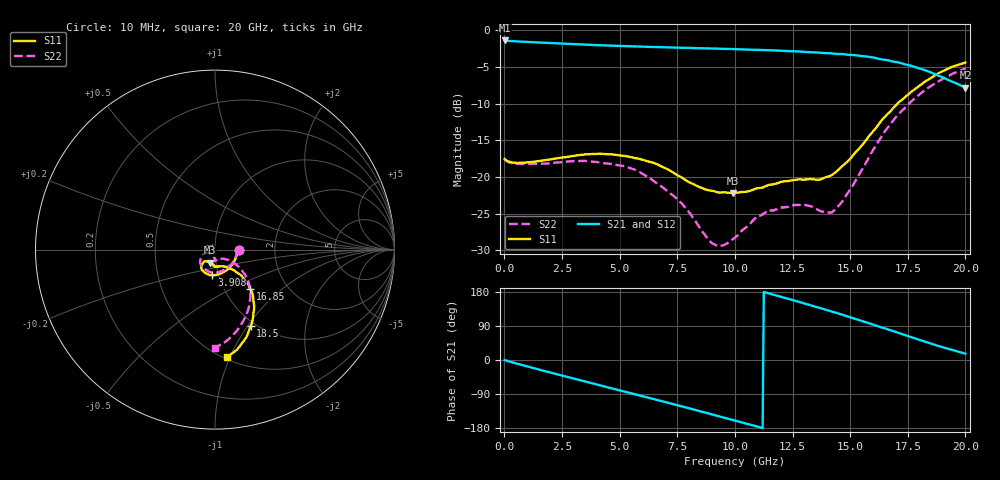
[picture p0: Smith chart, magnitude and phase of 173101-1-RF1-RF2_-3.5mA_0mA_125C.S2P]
!  2-Port S-parameters saved by WinCal
! VAR MeasName=S-Parameters (CALIBRATED_DATA) read from VNA (N5242A)
! VAR MeasDate=2017-7-20 10:59:46
! VAR NAME=173101-1-RF1-RF2_-3.5mA_0mA_125C
! VAR FILENAME=173101-1-RF1-RF2_-3.5mA_0mA_125C.S2P
! VAR DATE=2017-7-20 10:59:46
! VAR PHYS_PORTS=1,2
# Hz S DB R 50
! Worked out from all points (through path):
!   401 points, 10 MHz to 20 GHz, reference 50 ohm
!   highest |S21| = -1.40 dB at 10 MHz (marker M1); lowest = -7.8 dB at 20 GHz (marker M2)
!   group delay of S21, straight-line fit = 47.2 ps
!   lowest |S11| = -22.2 dB at 9.905 GHz (marker M3), VSWR 1.17, Z = 47 - j6.92 ohm
!   |S11| at or under -10 dB: start of sweep to 17.06 GHz
!   |S22| runs from -29.4 to -5.2 dB; largest |S21 - S12| = 0.0039
!   S11 on the Smith chart (normalised r, x): 10 MHz: 1.31, -0.01; 3.908 GHz: 0.92, -0.27; 16.85 GHz: 1.32, -0.63; 18.5 GHz: 0.94, -1.04; 20 GHz: 0.52, -0.98
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1e7  -17.57 -1.1  -1.40 -0.2  -1.40 -0.2  -17.57 -0.9
1.559225e9  -17.82 -48.7  -1.69 -26.2  -1.69 -26.2  -18.22 -50.8
3.358325e9  -16.99 -89.0  -1.96 -54.6  -1.96 -54.6  -17.80 -95.8
3.90805e9  -16.87 -97.8  -2.03 -63.1  -2.03 -63.2  -17.94 -106.7
5.357325e9  -17.21 -118.6  -2.19 -85.7  -2.20 -85.7  -18.69 -132.8
6.70665e9  -18.40 -128.9  -2.30 -106.8  -2.29 -106.7  -21.08 -150.1
7.70615e9  -20.11 -132.7  -2.40 -122.5  -2.41 -122.5  -23.66 -157.9
9.055475e9  -21.91 -123.6  -2.49 -144.1  -2.48 -144.1  -29.12 -140.3
9.455275e9  -22.12 -117.1  -2.54 -150.7  -2.53 -150.7  -29.38 -123.6
9.90505e9  -22.19 -109.6  -2.57 -158.1  -2.57 -158.1  -28.51 -107.7
1.0005e10  -22.16 -108.5  -2.59 -159.7  -2.59 -159.8  -28.28 -105.1
1.095452e10  -21.55 -98.5  -2.68 -175.4  -2.68 -175.4  -25.44 -89.6
1.165418e10  -21.03 -95.0  -2.75 172.7  -2.76 172.7  -24.52 -90.6
1.335332e10  -20.28 -81.0  -3.01 143.2  -2.99 143.3  -24.06 -89.3
1.410295e10  -19.91 -66.6  -3.14 129.7  -3.16 129.6  -24.90 -66.3
1.445278e10  -19.12 -60.5  -3.25 123.3  -3.24 123.4  -24.09 -54.7
1.570215e10  -14.92 -46.3  -3.59 99.2  -3.61 99.3  -17.97 -35.1
1.670165e10  -11.18 -46.8  -4.14 79.4  -4.17 79.1  -12.97 -40.5
1.685158e10  -10.69 -48.1  -4.26 76.4  -4.27 76.5  -12.40 -42.4
1.775112e10  -8.17 -56.1  -4.96 58.2  -4.97 58.2  -9.45 -54.4
1.850075e10  -6.53 -65.1  -5.76 43.3  -5.78 43.2  -7.62 -66.5
2e10  -4.39 -83.5  -7.82 16.6  -7.85 17.1  -5.24 -90.1
